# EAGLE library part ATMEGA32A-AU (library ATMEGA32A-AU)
8-bit Microcontroller
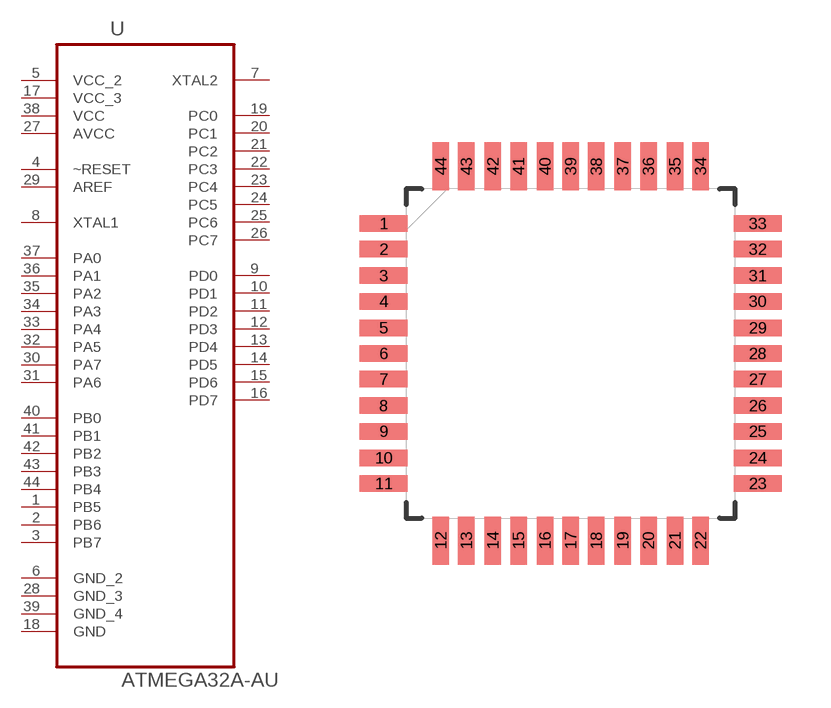
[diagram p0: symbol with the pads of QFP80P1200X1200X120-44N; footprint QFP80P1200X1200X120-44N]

Designator prefix U

## ATMEGA32A-AU (Availability: Unavailable; Description: AVR AVR® ATmega Microcontroller IC 8-Bit 16MHz 32KB _16K x 16_ FLASH 44-TQFP _10x10_; MF: Microchip; MP: ATMEGA32A-AU; Package: TQFP-44 Microchip; Price: None)  [QFP80P1200X1200X120-44N]
1  PB5
2  PB6
3  PB7
4  ~RESET  in
5  VCC_2  pwr
6  GND_2  pas
7  XTAL2  out
8  XTAL1  in
9  PD0
10  PD1
11  PD2
12  PD3
13  PD4
14  PD5
15  PD6
16  PD7
17  VCC_3  pwr
18  GND  pas
19  PC0
20  PC1
21  PC2
22  PC3
23  PC4
24  PC5
25  PC6
26  PC7
27  AVCC  pwr
28  GND_3  pas
29  AREF  in
30  PA7
31  PA6
32  PA5
33  PA4
34  PA3
35  PA2
36  PA1
37  PA0
38  VCC  pwr
39  GND_4  pas
40  PB0
41  PB1
42  PB2
43  PB3
44  PB4

## Footprint QFP80P1200X1200X120-44N (pad centres in mm)
smd 1.473 x 0.508: 1 -5.74,3.988; 2 -5.74,3.2; 3 -5.74,2.388; 4 -5.74,1.6; 5 -5.74,0.787; 6 -5.74,0; 7 -5.74,-0.787; 8 -5.74,-1.6; 9 -5.74,-2.388; 10 -5.74,-3.2; 11 -5.74,-3.988; 23 5.74,-3.988; 24 5.74,-3.2; 25 5.74,-2.388; 26 5.74,-1.6; 27 5.74,-0.787; 28 5.74,0; 29 5.74,0.787; 30 5.74,1.6; 31 5.74,2.388; 32 5.74,3.2; 33 5.74,3.988
smd 0.508 x 1.473: 12 -3.988,-5.74; 13 -3.2,-5.74; 14 -2.388,-5.74; 15 -1.6,-5.74; 16 -0.787,-5.74; 17 0,-5.74; 18 0.787,-5.74; 19 1.6,-5.74; 20 2.388,-5.74; 21 3.2,-5.74; 22 3.988,-5.74; 34 3.988,5.74; 35 3.2,5.74; 36 2.388,5.74; 37 1.6,5.74; 38 0.787,5.74; 39 0,5.74; 40 -0.787,5.74; 41 -1.6,5.74; 42 -2.388,5.74; 43 -3.2,5.74; 44 -3.988,5.74

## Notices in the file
This work is licensed under a Creative Commons Attribution-ShareAlike 4.0 International License (CC BY-SA) with Design Exception 1.0
